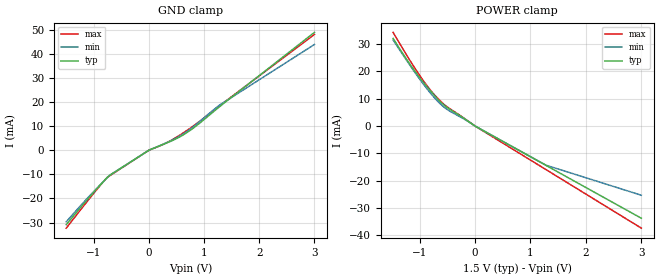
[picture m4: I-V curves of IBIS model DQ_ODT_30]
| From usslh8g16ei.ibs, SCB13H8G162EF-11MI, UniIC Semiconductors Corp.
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|   Model DQ_ODT_30
[Model] DQ_ODT_30
Model_type Input
Polarity   Non-Inverting
Enable   Active-High
Vinl =  0.615V
Vinh =  0.885V
C_comp   0.976pF   0.912pF   0.988pF
C_comp_power_clamp   0.637pF   0.566pF   0.642pF
C_comp_gnd_clamp   0.346pF   0.339pF   0.346pF
[Model Spec]
Vinh   0.885V   0.776V   0.922V
Vinl   0.615V   0.506V   0.652V
[Temperature Range]   45.000   95.000   -40.000
[Voltage Range]   1.500V   1.283V   1.575V
[C Comp Corner]
C_comp_power_clamp   0.642pF   0.566pF   0.637pF
C_comp_gnd_clamp   0.346pF   0.346pF   0.339pF
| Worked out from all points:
|   GND clamp passes 1 mA (typ) near -0.07 V on its own axis
|   POWER clamp passes 1 mA (typ) near -0.07 V on its own axis
[GND_clamp]
|Voltage   I(typ)   I(min)   I(max)
-1.5V     -30.89mA   -29.69mA   -32.31mA
-1.066V   -19.11mA   -18.69mA   -19.71mA
-756mV    -11.32mA   -11.38mA   -11.28mA
-694mV    -10.18mA   -10.13mA   -10.35mA
-12mV     -176uA     -175.2uA   -179uA
360mV     3.354mA    3.518mA    3.555mA
546mV     5.369mA    5.699mA    6.059mA
732mV     7.969mA    8.447mA    8.869mA
1.29V     18.2mA     18.83mA    18.59mA
3V        48.81mA    43.8mA     47.96mA
[POWER_clamp]
|Voltage   I(typ)   I(min)   I(max)
-1.476V   32.02mA    31.46mA    34.22mA
-1.166V   22.4mA     22.02mA    23.76mA
-887mV    14.87mA    14.17mA    15.31mA
-670mV    9.819mA    8.986mA    10.07mA
-484mV    6.509mA    5.813mA    6.738mA
12mV      -134.9uA   -134.2uA   -149.3uA
1.283V    -14.42mA   -14.35mA   -15.97mA
3V        -33.72mA   -25.31mA   -37.33mA
